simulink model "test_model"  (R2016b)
settings: Solver=VariableStepAuto  StartTime=0.0  StopTime=8.4  RelTol=1e-3
InitFcn:
  | clear mex
  | delete test_model_sfun.mexw64
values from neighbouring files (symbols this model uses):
  g = 9.81    [modelParameters.m]    (also in analyzeIMU_data.m = 9.8; getMomentOfInertia.m = 9.80665)
  height_controlled_o = (((Rm*If +      + (((omega_o * 2 * Rm * Kv * Kq       * Kd + 1)^2) - 1)/(4* Rm*Kv^2*Kq      *Kd))/Vb)*(Pmax- Pmin)+Pmin)    [modelParameters.m]
  If = 0.511    [modelParameters.m]    (also in thrustDragConstantCalculations.m = [If0; If1; If2; If3]; Kd_error.m = I_0 * sign(rotor_speed_0) + I_1 * rotor_speed_0 + I_2 * roto)
  Jreq = 4.2012e-05    [modelParameters.m]
  Jxx = 0.0130    (= 0.013)    [modelParameters.m]
  Jyy = 0.0140    (= 0.014)    [modelParameters.m]
  Jzz = 0.0285    [modelParameters.m]
  Kd = 1.0317e-7    (= 1.0317e-07)    [modelParameters.m]    (also in calcDragConstant.m = ((A'*A)^-1)*A'*b; thrustDragConstantCalculations.m = calcDragConstant(data, Pmin, Pmax, Rm, Kv, Kq, If); Kd_error.m)
  Kq = 96.3422    [modelParameters.m]    (also in thrustDragConstantCalculations.m; Kd_error.m)
  Kt = 8.6519e-6    (= 8.6519e-06)    [modelParameters.m]    (also in calcThrustConstant.m = ((A'*A)^(-1))*(A'*T); thrustDragConstantCalculations.m = calcThrustConstant(data))
  Kv = 96.3422    [modelParameters.m]    (also in thrustDragConstantCalculations.m; Kd_error.m)
  logAnalysisToggle = 1    [modelParameters.m]
  m = 1.244    [modelParameters.m]
  omega_o = sqrt((m*g)/(4*Kt))    [modelParameters.m]
  Pmax = 2e5    (= 200000)    [modelParameters.m]    (also in thrustDragConstantCalculations.m; Kd_error.m)
  Pmin = 1e5    (= 100000)    [modelParameters.m]    (also in thrustDragConstantCalculations.m; Kd_error.m)
  rhx = 0.16    [modelParameters.m]
  rhy = 0.16    [modelParameters.m]
  rhz = 0.03    [modelParameters.m]
  Rm = 0.2308    [modelParameters.m]    (also in thrustDragConstantCalculations.m; Kd_error.m)
  Tc = 0.04    [modelParameters.m]
  Tq = 0.005    [modelParameters.m]
  Vb = 11.1    [modelParameters.m]    (also in calcDragConstant.m = [data.(6); data.(6); data.(6); data.(6)]; Kd_error.m = data.(6))
  x_controlled_o = 0    [modelParameters.m]
  y_controlled_o = 0    [modelParameters.m]
  yaw_controlled_o = 0    [modelParameters.m]
undefined symbols (not defined in the file or in its folder): DiscIntNeverNeededParam
libraries: simulink x13, vrlib x2

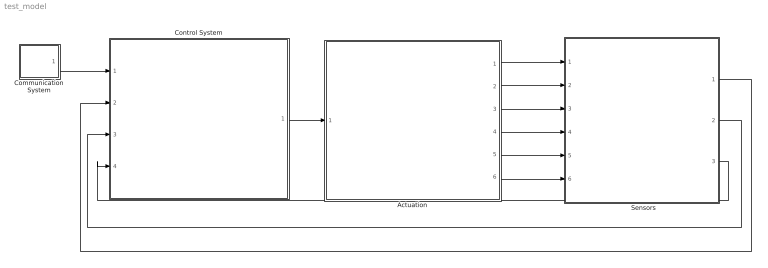
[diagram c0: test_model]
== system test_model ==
  "     Sensors   " : Subsystem
  Actuation : Subsystem
  Communication System : Subsystem
  Control System : Subsystem
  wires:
  Control System/1(P) -> Actuation/1(P)
  Communication System/1(setpoints) -> Control System/1(setpoints)
  Actuation/1(B_omega) -> "     Sensors   "/1(B_Omega)
  Actuation/2(euler_angles) -> "     Sensors   "/2(euler_angles)
  Actuation/3(B_vo) -> "     Sensors   "/3(B_vo)
  Actuation/4(E_ro) -> "     Sensors   "/4(E_ro)
  Actuation/5(B_vo_dot) -> "     Sensors   "/5(B_vo_dot)
  Actuation/6(B_g) -> "     Sensors   "/6(B_g)
  "     Sensors   "/3(current_position) -> Control System/4(current_position)
  "     Sensors   "/2(euler_rates) -> Control System/3(euler_rates)
  "     Sensors   "/1(euler_angles_filtered) -> Control System/2(euler_angles_filtered)

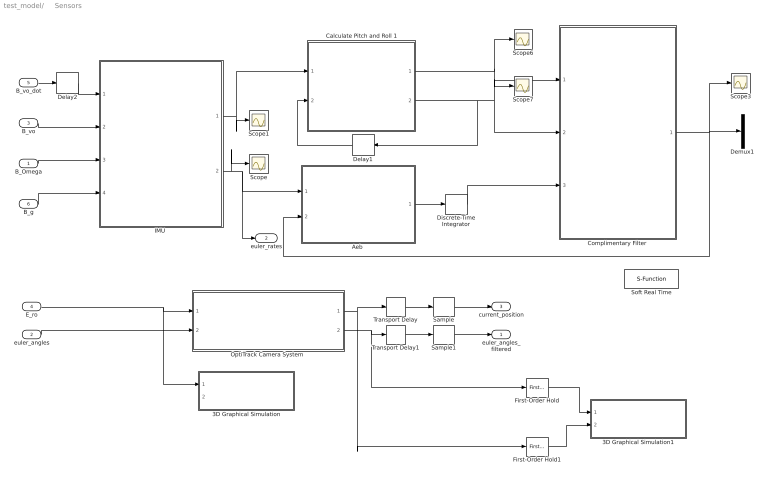
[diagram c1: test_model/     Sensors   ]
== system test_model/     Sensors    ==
  B_Omega : Inport
  euler_angles : Inport  Port=2
  B_vo : Inport  Port=3
  E_ro : Inport  Port=4
  B_vo_dot : Inport  Port=5
  B_g : Inport  Port=6
  3D Graphical Simulation : Subsystem  Commented=on
  3D Graphical Simulation1 : Subsystem  Commented=on
  "Aeb " : MATLAB Function  TreatAsAtomicUnit=on
  Calculate Pitch and Roll 1 : MATLAB Function  TreatAsAtomicUnit=on
  "Complimentary Filter " : MATLAB Function  TreatAsAtomicUnit=on
  Delay1 : Delay  DelayLength=1  InitialCondition=0  SampleTime=Tq
  Delay2 : Delay  DelayLength=1  InitialCondition=0  SampleTime=Tq
  Demux1 : Demux  Outputs=2
  Discrete-Time Integrator : DiscreteIntegrator  InitialConditionSetting=State (most efficient)  SampleTime=Tq  ICPrevOutput=DiscIntNeverNeededParam  ICPrevScaledInput=DiscIntNeverNeededParam
  First-Order Hold : simulink/Discrete/First-Order Hold  DisableCoverage=on  Ts=5e-3
  First-Order Hold1 : simulink/Discrete/First-Order Hold  DisableCoverage=on  Ts=5e-3
  "IMU " : Subsystem
  "OptiTrack Camera System " : Subsystem
  Sample : ZeroOrderHold  SampleTime=Tc
  Sample1 : ZeroOrderHold  SampleTime=Tc
  Scope{,1,3,6..7} (5 alike) : Scope
  Soft Real Time : S-Function  Commented=on  FunctionName=sfun_time  Parameters=x  SFunctionDeploymentMode=off  EnableBusSupport=off
  Transport Delay : TransportDelay  DelayTime=6e-3
  Transport Delay1 : TransportDelay  DelayTime=6e-3
  euler_angles_filtered : Outport
  euler_rates : Outport  Port=2
  current_position : Outport  Port=3
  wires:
  "IMU "/1(accelerometer) -> Calculate Pitch and Roll 1/1(accel_reading), Scope1/1
  "IMU "/2(gyroscope) -> Scope/1, euler_rates/1, "Aeb "/1(gyro_reading)
  B_vo/1 -> "IMU "/2(B_vo)
  B_Omega/1 -> "IMU "/3(B_Omega)
  B_g/1 -> "IMU "/4(B_g)
  Calculate Pitch and Roll 1/2(accel_roll) -> Scope7/1, "Complimentary Filter "/2(accel_roll), Delay1/1
  Calculate Pitch and Roll 1/1(accel_pitch) -> Scope6/1, "Complimentary Filter "/1(accel_pitch)
  Delay1/1 -> Calculate Pitch and Roll 1/2(accel_roll_prev)
  euler_angles/1 -> "OptiTrack Camera System "/2(yaw)
  First-Order Hold/1 -> 3D Graphical Simulation1/1("Euler Angles ")
  E_ro/1 -> 3D Graphical Simulation/1(Displacement), "OptiTrack Camera System "/1(E_ro)
  First-Order Hold1/1 -> 3D Graphical Simulation1/2(Displacement)
  B_vo_dot/1 -> Delay2/1
  Delay2/1 -> "IMU "/1(B_vo_dot)
  "Aeb "/1(euler_rates_IMU) -> Discrete-Time Integrator/1
  Discrete-Time Integrator/1 -> "Complimentary Filter "/3(euler_angles_gyro)
  "OptiTrack Camera System "/1(E_ro_camera) -> Transport Delay/1, First-Order Hold1/1
  "OptiTrack Camera System "/2(yaw_camera) -> First-Order Hold/1, Transport Delay1/1
  Transport Delay/1 -> Sample/1
  Transport Delay1/1 -> Sample1/1
  Sample/1 -> current_position/1
  Sample1/1 -> euler_angles_filtered/1
  "Complimentary Filter "/1(euler_angles_IMU) -> "Aeb "/2(euler_angles_IMU), Scope3/1, Demux1/1

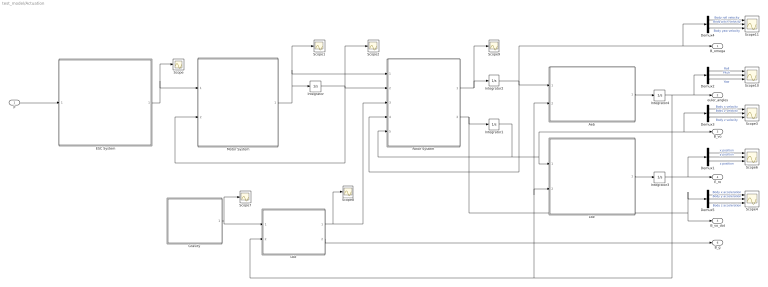
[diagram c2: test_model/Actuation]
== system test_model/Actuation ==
  P : Inport
  "Aeb " : MATLAB Function  TreatAsAtomicUnit=on
  Demux{1..5} (5 alike) : Demux  Outputs=3
  ESC System : MATLAB Function  TreatAsAtomicUnit=on
  "Gravity " : MATLAB Function  TreatAsAtomicUnit=on
  Integrator : Integrator  InitialCondition=[omega_o, omega_o, omega_o, omega_o]
  Integrator1 : Integrator  InitialCondition=[0; 0; 0]
  Integrator2 : Integrator  InitialCondition=[0; 0; 0]
  Integrator3 : Integrator  InitialCondition=[0; 0; 0]
  Integrator4 : Integrator  InitialCondition=[0; 0; 0]  ContinuousStateAttributes=['phi' 'theta' 'psi']
  "Lbe " : MATLAB Function  TreatAsAtomicUnit=on
  "Lbe " : MATLAB Function  TreatAsAtomicUnit=on
  Motor System : MATLAB Function  TreatAsAtomicUnit=on
  "Rotor System " : MATLAB Function  TreatAsAtomicUnit=on
  Scope{,1..2,7..9} (6 alike) : Scope
  Scope{3..4,6,10..11} (5 alike) : Scope  NumInputPorts=3
  B_omega : Outport
  euler_angles : Outport  Port=2
  B_vo : Outport  Port=3
  E_ro : Outport  Port=4
  B_vo_dot : Outport  Port=5
  B_g : Outport  Port=6
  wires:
  ESC System/1(Vb_eff) -> Scope/1, Motor System/1(Vb_eff)
  Motor System/1(w_dot) -> Integrator/1, "Rotor System "/1(w_dot), Scope1/1
  Integrator/1 -> Motor System/2(w), "Rotor System "/2(w), Scope2/1
  "Rotor System "/1(B_omega_dot) -> Scope9/1, Integrator2/1
  Integrator2/1 -> "Rotor System "/4(B_omega), B_omega/1, Demux4/1, "Aeb "/1(B_omega)
  "Aeb "/1(euler_rates) -> Integrator4/1
  "Gravity "/1(E_Fg) -> Scope7/1, "Lbe "/1(E_Fg)
  "Lbe "/1(E_ro) -> Integrator3/1
  Integrator3/1 -> Demux1/1, E_ro/1
  "Lbe "/1(B_Fg) -> Scope8/1, "Rotor System "/3(B_Fg)
  "Lbe "/2(B_g) -> B_g/1
  Demux1/2 -> Scope6/2  "y position"
  Demux1/1 -> Scope6/1  "x position"
  Demux1/3 -> Scope6/3  "z position"
  Demux2/2 -> Scope10/2  "Pitch"
  Demux2/1 -> Scope10/1  "Roll"
  Demux2/3 -> Scope10/3  "Yaw"
  Demux4/2 -> Scope11/2  "Body pitch velocity"
  Demux4/1 -> Scope11/1  "Body roll velocity"
  Demux4/3 -> Scope11/3  "Body yaw velocity"
  Demux3/2 -> Scope3/2  "Body y velocity"
  Demux3/1 -> Scope3/1  "Body x velocity"
  Demux3/3 -> Scope3/3  "Body z velocity"
  Demux5/2 -> Scope4/2  "Body y acceleration"
  Demux5/1 -> Scope4/1  "Body x acceleration"
  Demux5/3 -> Scope4/3  "Body z acceleration"
  Integrator1/1 -> "Rotor System "/5(B_vo), "Lbe "/1(B_vo), Demux3/1, B_vo/1
  "Rotor System "/2(B_vo_dot) -> Demux5/1, B_vo_dot/1, Integrator1/1
  Integrator4/1 -> euler_angles/1, Demux2/1, "Lbe "/2(euler_angles), "Aeb "/2(euler_angles), "Lbe "/2(euler_angles)
  P/1 -> ESC System/1(P)

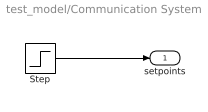
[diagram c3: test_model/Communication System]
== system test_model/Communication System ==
  Step : Step  Before=[0; 0; 0; 0]  After=[1; 1; 0; 0]  SampleTime=Tq
  setpoints : Outport
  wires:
  Step/1 -> setpoints/1

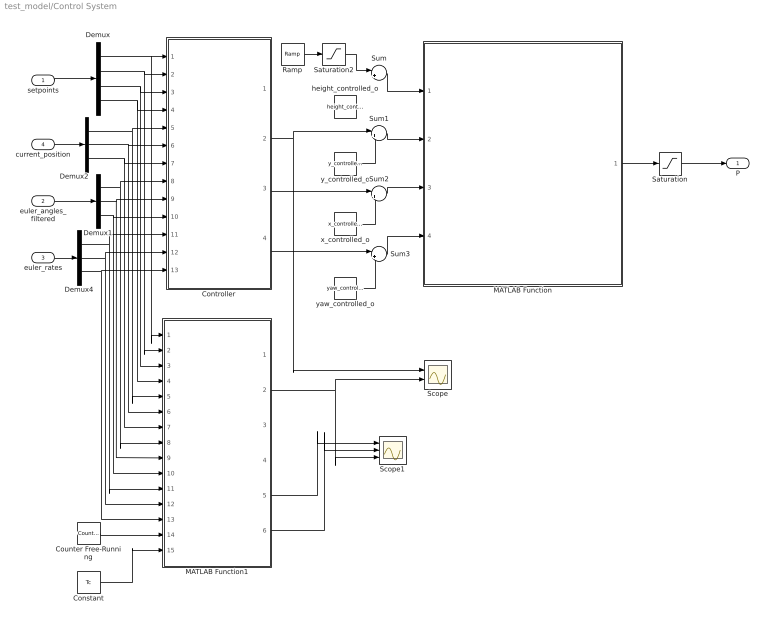
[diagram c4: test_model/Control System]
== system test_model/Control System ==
  setpoints : Inport
  euler_angles_filtered : Inport  Port=2
  euler_rates : Inport  Port=3
  current_position : Inport  Port=4
  Constant : Constant  Value=Tc  SampleTime=Tc
  Controller : Subsystem
  Counter Free-Running : simulink/Sources/Counter Free-Running  NumBits=32  tsamp=Tc
  Demux : Demux
  Demux1 : Demux  Outputs=3
  Demux2 : Demux  Outputs=3
  Demux4 : Demux  Outputs=3
  MATLAB Function : MATLAB Function  TreatAsAtomicUnit=on
  MATLAB Function1 : MATLAB Function  TreatAsAtomicUnit=on  SystemSampleTime=Tq
  Ramp : simulink/Sources/Ramp  slope=height_controlled_o  start=6.32  X0=0
  Saturation : Saturate  UpperLimit=Pmax*ones(4,1)  LowerLimit=Pmin*ones(4,1)
  Saturation2 : Saturate  UpperLimit=height_controlled_o  LowerLimit=0
  Scope : Scope  NumInputPorts=2
  Scope1 : Scope  NumInputPorts=3
  Sum{,1..3} (4 alike) : Sum  Inputs=|++
  height_controlled_o : Constant  Value=height_controlled_o  SampleTime=Tc
  x_controlled_o : Constant  Value=x_controlled_o
  y_controlled_o : Constant  Value=y_controlled_o
  yaw_controlled_o : Constant  Value=yaw_controlled_o
  P : Outport
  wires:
  setpoints/1 -> Demux/1
  euler_angles_filtered/1 -> Demux1/1
  current_position/1 -> Demux2/1
  euler_rates/1 -> Demux4/1
  Demux/1 -> MATLAB Function1/1(set_x), Controller/1(x_setpoint)
  Demux/2 -> MATLAB Function1/2(set_y), Controller/2(y_setpoint)
  Demux/3 -> MATLAB Function1/3(set_z), Controller/3(z_setpoint)
  Demux2/1 -> MATLAB Function1/5(cur_x), Controller/5(x_position)
  Demux2/2 -> Controller/6(y_position), MATLAB Function1/6(cur_y)
  Demux2/3 -> MATLAB Function1/7(cur_z), Controller/7(z_position)
  Controller/2(y_controlled) -> Scope/1, Sum1/1
  Controller/4(yaw_controlled) -> Sum3/1
  y_controlled_o/1 -> Sum1/2
  x_controlled_o/1 -> Sum2/2
  yaw_controlled_o/1 -> Sum3/2
  MATLAB Function/1(P) -> Saturation/1
  Demux1/1 -> Controller/8(roll), MATLAB Function1/8(cur_phi)
  Demux1/2 -> MATLAB Function1/9(cur_theta), Controller/9(pitch)
  Demux4/1 -> Controller/11(roll_rate), MATLAB Function1/11(cur_phi_d)
  Demux4/2 -> Controller/12(pitch_rate), MATLAB Function1/12(cur_theta_d)
  Demux4/3 -> MATLAB Function1/13(cur_psi_d), Controller/13(yaw_rate)
  Demux/4 -> MATLAB Function1/4(set_yaw), Controller/4(yaw_setpoint)
  Demux1/3 -> MATLAB Function1/10(cur_psi), Controller/10(yaw)
  Controller/3(x_controlled) -> Sum2/1
  Counter Free-Running/1 -> MATLAB Function1/14(vrpn_id)
  Saturation/1 -> P/1
  Constant/1 -> MATLAB Function1/15(Tc)
  Sum3/1 -> MATLAB Function/4(yaw_controlled)
  Sum2/1 -> MATLAB Function/3(x_controlled)
  Sum1/1 -> MATLAB Function/2(y_controlled)
  Sum/1 -> MATLAB Function/1(height_controlled)
  MATLAB Function1/5(pid_y_out) -> Scope1/1
  MATLAB Function1/6(pid_roll_out) -> Scope1/2
  MATLAB Function1/2(y_cor) -> Scope1/3, Scope/2
  Saturation2/1 -> Sum/1
  Ramp/1 -> Saturation2/1

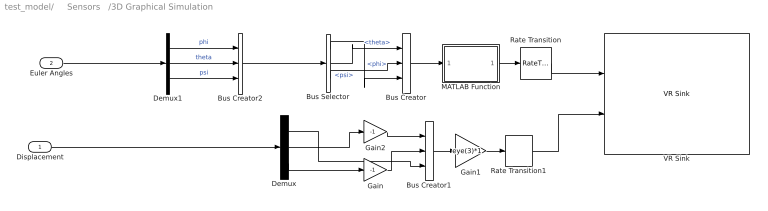
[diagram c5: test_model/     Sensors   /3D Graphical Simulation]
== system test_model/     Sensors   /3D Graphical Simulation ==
  Displacement : Inport
  Euler Angles : Inport  Port=2
  Bus Creator : BusCreator  Inputs=3
  Bus Creator1 : BusCreator  Inputs=3
  Bus Creator2 : BusCreator  Inputs=3
  Bus Selector : BusSelector  OutputSignals=phi,theta,psi
  Demux : Demux  Outputs=3
  Demux1 : Demux  Outputs=3
  Gain : Gain  Gain=-1
  Gain1 : Gain  Gain=eye(3)*1  Multiplication=Matrix(K*u)
  Gain2 : Gain  Gain=-1
  MATLAB Function : MATLAB Function  TreatAsAtomicUnit=on
  Rate Transition : RateTransition  OutPortSampleTime=0.06
  Rate Transition1 : RateTransition  OutPortSampleTime=0.06
  VR Sink : vrlib/VR Sink  InstantiateOnLoad=on  SampleTime=-1  ViewEnable=on  RemoteChange=off  RemoteView=off  FieldsWritten=Helicopter.rotation.4.1.1.double#Helicopter.translation.3.1.1.double  WorldFileName=quadrotor_world_ucart.wrl  AutoView=on  VideoDimensions=[]  AllowVariableSize=off
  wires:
  Displacement/1 -> Demux/1
  Bus Creator2/1 -> Bus Selector/1
  Demux/1 -> Bus Creator1/3
  Gain/1 -> Bus Creator1/2
  Gain2/1 -> Bus Creator1/1
  Rate Transition1/1 -> VR Sink/2
  Rate Transition/1 -> VR Sink/1
  Demux/3 -> Gain/1
  Demux/2 -> Gain2/1
  Bus Creator1/1 -> Gain1/1
  Bus Selector/1 -> Bus Creator/3  "<phi>"
  Bus Selector/3 -> Bus Creator/2  "<psi>"
  Bus Selector/2 -> Bus Creator/1  "<theta>"
  Gain1/1 -> Rate Transition1/1
  Demux1/3 -> Bus Creator2/3  "psi"
  Demux1/2 -> Bus Creator2/2  "theta"
  Demux1/1 -> Bus Creator2/1  "phi"
  Euler Angles/1 -> Demux1/1
  Bus Creator/1 -> MATLAB Function/1(u)
  MATLAB Function/1(y) -> Rate Transition/1

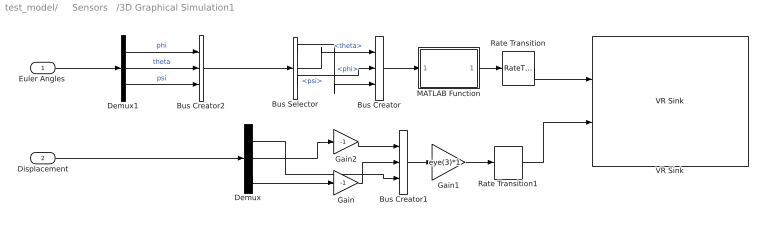
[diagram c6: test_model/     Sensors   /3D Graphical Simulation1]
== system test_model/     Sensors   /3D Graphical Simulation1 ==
  "Euler Angles " : Inport
  Displacement : Inport  Port=2
  Bus Creator : BusCreator  Inputs=3
  Bus Creator1 : BusCreator  Inputs=3
  Bus Creator2 : BusCreator  Inputs=3
  Bus Selector : BusSelector  OutputSignals=phi,theta,psi
  Demux : Demux  Outputs=3
  Demux1 : Demux  Outputs=3
  Gain : Gain  Gain=-1
  Gain1 : Gain  Gain=eye(3)*1  Multiplication=Matrix(K*u)
  Gain2 : Gain  Gain=-1
  MATLAB Function : MATLAB Function  TreatAsAtomicUnit=on
  Rate Transition : RateTransition  OutPortSampleTime=0.06
  Rate Transition1 : RateTransition  OutPortSampleTime=0.06
  VR Sink : vrlib/VR Sink  InstantiateOnLoad=on  SampleTime=-1  ViewEnable=on  RemoteChange=off  RemoteView=off  FieldsWritten=Helicopter.rotation.4.1.1.double#Helicopter.translation.3.1.1.double  WorldFileName=quadrotor_world_ucart.wrl  AutoView=on  VideoDimensions=[]  AllowVariableSize=off
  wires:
  Bus Creator2/1 -> Bus Selector/1
  Demux/1 -> Bus Creator1/3
  Gain/1 -> Bus Creator1/2
  Gain2/1 -> Bus Creator1/1
  Rate Transition1/1 -> VR Sink/2
  Rate Transition/1 -> VR Sink/1
  Demux/3 -> Gain/1
  Demux/2 -> Gain2/1
  Bus Creator1/1 -> Gain1/1
  Bus Selector/1 -> Bus Creator/3  "<phi>"
  Bus Selector/3 -> Bus Creator/2  "<psi>"
  Bus Selector/2 -> Bus Creator/1  "<theta>"
  Gain1/1 -> Rate Transition1/1
  Demux1/3 -> Bus Creator2/3  "psi"
  Demux1/2 -> Bus Creator2/2  "theta"
  Demux1/1 -> Bus Creator2/1  "phi"
  Bus Creator/1 -> MATLAB Function/1(u)
  MATLAB Function/1(y) -> Rate Transition/1
  Displacement/1 -> Demux/1
  "Euler Angles "/1 -> Demux1/1

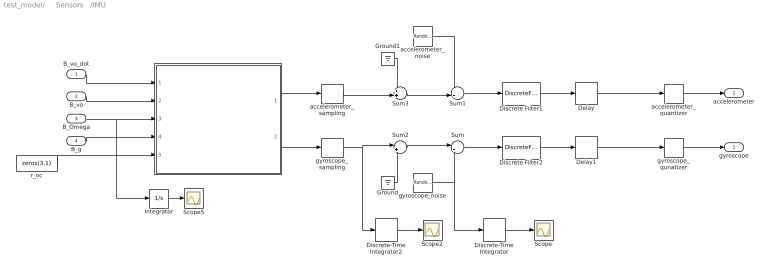
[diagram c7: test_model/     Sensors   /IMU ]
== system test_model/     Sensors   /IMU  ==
  B_vo_dot : Inport
  B_vo : Inport  Port=2
  B_Omega : Inport  Port=3
  B_g : Inport  Port=4
  " " : MATLAB Function  TreatAsAtomicUnit=on
  Delay : Delay  DelayLength=4  InitialCondition=0  SampleTime=Tq
  Delay1 : Delay  DelayLength=4  InitialCondition=0  SampleTime=Tq
  Discrete Filter1 : DiscreteFilter  Numerator=[0 0.1454]  Denominator=[1 -0.8546]  SampleTime=Tq
  Discrete Filter2 : DiscreteFilter  Numerator=[0 0.1454]  Denominator=[1 -0.8546]  SampleTime=Tq
  Discrete-Time Integrator : DiscreteIntegrator  InitialConditionSetting=State (most efficient)  SampleTime=-1  ICPrevOutput=DiscIntNeverNeededParam  ICPrevScaledInput=DiscIntNeverNeededParam
  Discrete-Time Integrator2 : DiscreteIntegrator  InitialConditionSetting=State (most efficient)  SampleTime=-1  ICPrevOutput=DiscIntNeverNeededParam  ICPrevScaledInput=DiscIntNeverNeededParam
  Ground : Ground
  Ground1 : Ground
  Integrator : Integrator
  Scope : Scope
  Scope2 : Scope
  Scope5 : Scope
  Sum : Sum  Inputs=|++
  Sum1 : Sum  Inputs=++|
  Sum2 : Sum  Inputs=|++
  Sum3 : Sum  Inputs=++|
  accelerometer_noise : RandomNumber  Mean=zeros(3,1)  Variance=[ 3e-7 ; 3.3e-7 ; 7.2e-7 ]  Seed=[0,1,2]  SampleTime=Tq
  accelerometer_quantizer : Quantizer  QuantizationInterval=2.4400e-04
  accelerometer_sampling : ZeroOrderHold  SampleTime=Tq
  gyroscope_noise : RandomNumber  Mean=zeros(3,1)  Variance=[ 2.2e-8 ; 1.1e-7 ; 2.4e-8 ]  Seed=[0,1,2]  SampleTime=Tq
  gyroscope_qunatizer : Quantizer  QuantizationInterval=1.1e-3
  gyroscope_sampling : ZeroOrderHold  SampleTime=Tq
  r_oc : Constant  Value=zeros(3,1)
  accelerometer : Outport
  gyroscope : Outport  Port=2
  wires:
  accelerometer_noise/1 -> Sum1/1
  Sum/1 -> Discrete Filter2/1
  Sum2/1 -> Sum/1
  Sum3/1 -> Sum1/2
  gyroscope_noise/1 -> Sum/2, Discrete-Time Integrator/1
  Sum1/1 -> Discrete Filter1/1
  gyroscope_sampling/1 -> Sum2/1, Discrete-Time Integrator2/1
  accelerometer_sampling/1 -> Sum3/2
  Ground/1 -> Sum2/2
  Ground1/1 -> Sum3/1
  B_vo_dot/1 -> " "/1(B_vo_dot)
  B_vo/1 -> " "/2(B_vo)
  B_Omega/1 -> Integrator/1, " "/3(B_Omega)
  B_g/1 -> " "/4(B_g)
  r_oc/1 -> " "/5(r_oc)
  " "/2(gyroReading) -> gyroscope_sampling/1
  " "/1(accelReading) -> accelerometer_sampling/1
  Discrete-Time Integrator/1 -> Scope/1
  Discrete-Time Integrator2/1 -> Scope2/1
  Integrator/1 -> Scope5/1
  gyroscope_qunatizer/1 -> gyroscope/1
  accelerometer_quantizer/1 -> accelerometer/1
  Discrete Filter2/1 -> Delay1/1
  Discrete Filter1/1 -> Delay/1
  Delay/1 -> accelerometer_quantizer/1
  Delay1/1 -> gyroscope_qunatizer/1

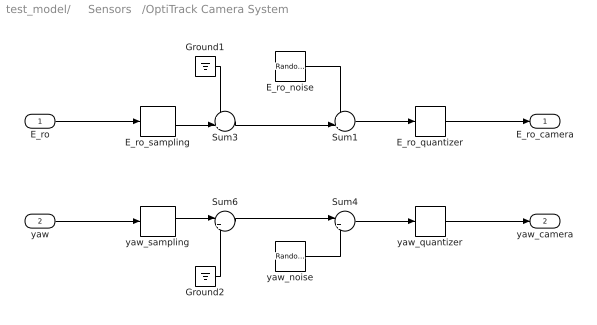
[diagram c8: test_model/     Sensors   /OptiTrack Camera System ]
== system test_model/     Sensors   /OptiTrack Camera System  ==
  E_ro : Inport
  yaw : Inport  Port=2
  E_ro_noise : RandomNumber  Mean=zeros(3,1)  Variance=[ 7.9664e-10 ; 1.1928e-10 ; 5.0636e-10 ]  Seed=[0,1,2]  SampleTime=Tc
  E_ro_quantizer : Quantizer  QuantizationInterval=2.4400e-04
  E_ro_sampling : ZeroOrderHold  SampleTime=Tc
  Ground1 : Ground
  Ground2 : Ground
  Sum1 : Sum  Inputs=++|
  Sum3 : Sum  Inputs=++|
  Sum4 : Sum  Inputs=|++
  Sum6 : Sum  Inputs=|++
  yaw_noise : RandomNumber  Variance=1.0783e-9  SampleTime=Tc
  yaw_quantizer : Quantizer  QuantizationInterval=1.1e-3
  yaw_sampling : ZeroOrderHold  SampleTime=Tc
  E_ro_camera : Outport
  yaw_camera : Outport  Port=2
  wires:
  E_ro_noise/1 -> Sum1/1
  Sum3/1 -> Sum1/2
  Sum1/1 -> E_ro_quantizer/1
  E_ro_sampling/1 -> Sum3/2
  Ground1/1 -> Sum3/1
  Sum4/1 -> yaw_quantizer/1
  Sum6/1 -> Sum4/1
  yaw_noise/1 -> Sum4/2
  yaw_sampling/1 -> Sum6/1
  Ground2/1 -> Sum6/2
  yaw/1 -> yaw_sampling/1
  E_ro/1 -> E_ro_sampling/1
  E_ro_quantizer/1 -> E_ro_camera/1
  yaw_quantizer/1 -> yaw_camera/1

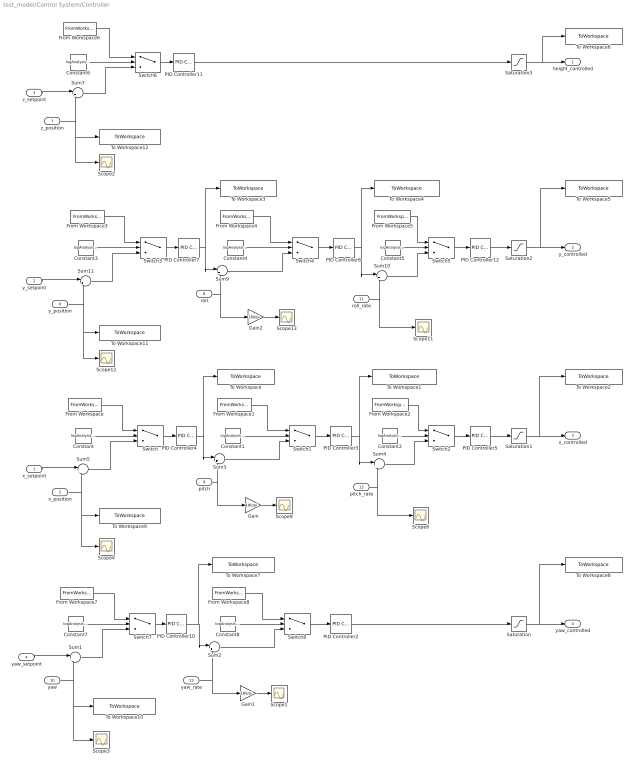
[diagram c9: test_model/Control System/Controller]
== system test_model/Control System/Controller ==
  x_setpoint : Inport
  y_setpoint : Inport  Port=2
  z_setpoint : Inport  Port=3
  yaw_setpoint : Inport  Port=4
  x_position : Inport  Port=5
  y_position : Inport  Port=6
  z_position : Inport  Port=7
  roll : Inport  Port=8
  pitch : Inport  Port=9
  yaw : Inport  Port=10
  roll_rate : Inport  Port=11
  pitch_rate : Inport  Port=12
  yaw_rate : Inport  Port=13
  Constant{,1..8} (9 alike) : Constant  Value=logAnalysisToggle
  From Workspace : FromWorkspace  VariableName=x_error  SampleTime=Tc
  From Workspace1 : FromWorkspace  VariableName=pitch_error  SampleTime=Tc
  From Workspace2 : FromWorkspace  VariableName=pitchrate_error  SampleTime=Tq
  From Workspace3 : FromWorkspace  VariableName=y_error  SampleTime=Tc
  From Workspace4 : FromWorkspace  VariableName=roll_error  SampleTime=Tc
  From Workspace5 : FromWorkspace  VariableName=rollrate_error  SampleTime=Tq
  From Workspace6 : FromWorkspace  VariableName=z_error  SampleTime=Tc
  From Workspace7 : FromWorkspace  VariableName=yaw_error  SampleTime=Tc
  From Workspace8 : FromWorkspace  VariableName=yawrate_error  SampleTime=Tc
  Gain : Gain  Gain=180/pi
  Gain1 : Gain  Gain=180/pi
  Gain2 : Gain  Gain=180/pi
  PID Controller10 : simulink/Continuous/PID Controller  Controller=PD  TimeDomain=Discrete-time  SampleTime=Tc  IntegratorMethod=Forward Euler  FilterMethod=Forward Euler  Form=Parallel  UseFilter=on  ControllerParametersSource=internal  P=4.73868196952772  I=2.36803176515497  D=1.0129554639517  N=3.83298618768959  InitialConditionSource=internal  InitialConditionForIntegrator=0  InitialConditionForFilter=0  ExternalReset=none  LimitOutput=off  UpperSaturationLimit=inf  LowerSaturationLimit=-inf  LinearizeAsGain=on  AntiWindupMode=none  Kb=1  TrackingMode=off  Kt=1  PParamMin=[]  PParamMax=[]  IParamMin=[]  IParamMax=[]  DParamMin=[]  DParamMax=[]  NParamMin=[]  NParamMax=[]  KbParamMin=[]  KbParamMax=[]  KtParamMin=[]  KtParamMax=[]  POutMin=[]  POutMax=[]  IOutMin=[]  IOutMax=[]  DOutMin=[]  DOutMax=[]  NOutMin=[]  NOutMax=[]  KbOutMin=[]  KbOutMax=[]  KtOutMin=[]  KtOutMax=[]  IntegratorOutMin=[]  IntegratorOutMax=[]  FilterOutMin=[]  FilterOutMax=[]  SumOutMin=[]  SumOutMax=[]  SumI1OutMin=[]  SumI1OutMax=[]  SumI2OutMin=[]  SumI2OutMax=[]  SumI3OutMin=[]  SumI3OutMax=[]  SumDOutMin=[]  SumDOutMax=[]  SaturationOutMin=[]  SaturationOutMax=[]  IntegratorContinuousStateAttributes=''  IntegratorStateMustResolveToSignalObject=off  IntegratorRTWStateStorageClass=Auto  FilterContinuousStateAttributes=''  FilterStateMustResolveToSignalObject=off  FilterRTWStateStorageClass=Auto  DifferentiatorICPrevScaledInput=0  DifferentiatorOutMin=[]  DifferentiatorOutMax=[]
  PID Controller11 : simulink/Continuous/PID Controller  Controller=PID  TimeDomain=Discrete-time  SampleTime=Tc  IntegratorMethod=Forward Euler  FilterMethod=Forward Euler  Form=Parallel  UseFilter=off  ControllerParametersSource=internal  P=-3138.91816077077  I=-320.189162634817  D=-7421.98260028101  N=5.79502261645411  InitialConditionSource=internal  InitialConditionForIntegrator=0  InitialConditionForFilter=0  ExternalReset=none  LimitOutput=off  UpperSaturationLimit=inf  LowerSaturationLimit=-inf  LinearizeAsGain=on  AntiWindupMode=none  Kb=1  TrackingMode=off  Kt=1  PParamMin=[]  PParamMax=[]  IParamMin=[]  IParamMax=[]  DParamMin=[]  DParamMax=[]  NParamMin=[]  NParamMax=[]  KbParamMin=[]  KbParamMax=[]  KtParamMin=[]  KtParamMax=[]  POutMin=[]  POutMax=[]  IOutMin=[]  IOutMax=[]  DOutMin=[]  DOutMax=[]  NOutMin=[]  NOutMax=[]  KbOutMin=[]  KbOutMax=[]  KtOutMin=[]  KtOutMax=[]  IntegratorOutMin=[]  IntegratorOutMax=[]  FilterOutMin=[]  FilterOutMax=[]  SumOutMin=[]  SumOutMax=[]  SumI1OutMin=[]  SumI1OutMax=[]  SumI2OutMin=[]  SumI2OutMax=[]  SumI3OutMin=[]  SumI3OutMax=[]  SumDOutMin=[]  SumDOutMax=[]  SaturationOutMin=[]  SaturationOutMax=[]  IntegratorContinuousStateAttributes=''  IntegratorStateMustResolveToSignalObject=off  IntegratorRTWStateStorageClass=Auto  FilterContinuousStateAttributes=''  FilterStateMustResolveToSignalObject=off  FilterRTWStateStorageClass=Auto  DifferentiatorICPrevScaledInput=0  DifferentiatorOutMin=[]  DifferentiatorOutMax=[]
  PID Controller12 : simulink/Continuous/PID Controller  Controller=P  TimeDomain=Discrete-time  SampleTime=Tq  IntegratorMethod=Forward Euler  FilterMethod=Forward Euler  Form=Parallel  UseFilter=off  ControllerParametersSource=internal  P=1835.12180866282  I=1575.82088970639  D=550  N=244.660686071579  InitialConditionSource=internal  InitialConditionForIntegrator=0  InitialConditionForFilter=0  ExternalReset=none  LimitOutput=off  UpperSaturationLimit=inf  LowerSaturationLimit=-inf  LinearizeAsGain=on  AntiWindupMode=none  Kb=1  TrackingMode=off  Kt=1  PParamMin=[]  PParamMax=[]  IParamMin=[]  IParamMax=[]  DParamMin=[]  DParamMax=[]  NParamMin=[]  NParamMax=[]  KbParamMin=[]  KbParamMax=[]  KtParamMin=[]  KtParamMax=[]  POutMin=[]  POutMax=[]  IOutMin=[]  IOutMax=[]  DOutMin=[]  DOutMax=[]  NOutMin=[]  NOutMax=[]  KbOutMin=[]  KbOutMax=[]  KtOutMin=[]  KtOutMax=[]  IntegratorOutMin=[]  IntegratorOutMax=[]  FilterOutMin=[]  FilterOutMax=[]  SumOutMin=[]  SumOutMax=[]  SumI1OutMin=[]  SumI1OutMax=[]  SumI2OutMin=[]  SumI2OutMax=[]  SumI3OutMin=[]  SumI3OutMax=[]  SumDOutMin=[]  SumDOutMax=[]  SaturationOutMin=[]  SaturationOutMax=[]  IntegratorContinuousStateAttributes=''  IntegratorStateMustResolveToSignalObject=off  IntegratorRTWStateStorageClass=Auto  FilterContinuousStateAttributes=''  FilterStateMustResolveToSignalObject=off  FilterRTWStateStorageClass=Auto  DifferentiatorICPrevScaledInput=0  DifferentiatorOutMin=[]  DifferentiatorOutMax=[]
  PID Controller2 : simulink/Continuous/PID Controller  Controller=P  TimeDomain=Discrete-time  SampleTime=Tc  IntegratorMethod=Forward Euler  FilterMethod=Forward Euler  Form=Parallel  UseFilter=on  ControllerParametersSource=internal  P=10205.7985086303  I=-77.7  D=2.32  N=1/0.0818  InitialConditionSource=internal  InitialConditionForIntegrator=0  InitialConditionForFilter=0  ExternalReset=none  ZeroCross=off  LimitOutput=off  UpperSaturationLimit=inf  LowerSaturationLimit=-inf  LinearizeAsGain=on  AntiWindupMode=none  Kb=1  TrackingMode=off  Kt=1  PParamMin=[]  PParamMax=[]  IParamMin=[]  IParamMax=[]  DParamMin=[]  DParamMax=[]  NParamMin=[]  NParamMax=[]  KbParamMin=[]  KbParamMax=[]  KtParamMin=[]  KtParamMax=[]  POutMin=[]  POutMax=[]  IOutMin=[]  IOutMax=[]  DOutMin=[]  DOutMax=[]  NOutMin=[]  NOutMax=[]  KbOutMin=[]  KbOutMax=[]  KtOutMin=[]  KtOutMax=[]  IntegratorOutMin=[]  IntegratorOutMax=[]  FilterOutMin=[]  FilterOutMax=[]  SumOutMin=[]  SumOutMax=[]  SumI1OutMin=[]  SumI1OutMax=[]  SumI2OutMin=[]  SumI2OutMax=[]  SumI3OutMin=[]  SumI3OutMax=[]  SumDOutMin=[]  SumDOutMax=[]  SaturationOutMin=[]  SaturationOutMax=[]  IntegratorContinuousStateAttributes=''  IntegratorStateMustResolveToSignalObject=off  IntegratorRTWStateStorageClass=Auto  FilterContinuousStateAttributes=''  FilterStateMustResolveToSignalObject=off  FilterRTWStateStorageClass=Auto  DifferentiatorICPrevScaledInput=0  DifferentiatorOutMin=[]  DifferentiatorOutMax=[]
  PID Controller3 : simulink/Continuous/PID Controller  Controller=P  TimeDomain=Discrete-time  SampleTime=Tc  IntegratorMethod=Forward Euler  FilterMethod=Forward Euler  Form=Parallel  UseFilter=off  ControllerParametersSource=internal  P=1  I=35.1207902652377  D=0.2  N=40.0107970227961  InitialConditionSource=internal  InitialConditionForIntegrator=0  InitialConditionForFilter=0  ExternalReset=none  LimitOutput=off  UpperSaturationLimit=inf  LowerSaturationLimit=-inf  LinearizeAsGain=on  AntiWindupMode=none  Kb=1  TrackingMode=off  Kt=1  PParamMin=[]  PParamMax=[]  IParamMin=[]  IParamMax=[]  DParamMin=[]  DParamMax=[]  NParamMin=[]  NParamMax=[]  KbParamMin=[]  KbParamMax=[]  KtParamMin=[]  KtParamMax=[]  POutMin=[]  POutMax=[]  IOutMin=[]  IOutMax=[]  DOutMin=[]  DOutMax=[]  NOutMin=[]  NOutMax=[]  KbOutMin=[]  KbOutMax=[]  KtOutMin=[]  KtOutMax=[]  IntegratorOutMin=[]  IntegratorOutMax=[]  FilterOutMin=[]  FilterOutMax=[]  SumOutMin=[]  SumOutMax=[]  SumI1OutMin=[]  SumI1OutMax=[]  SumI2OutMin=[]  SumI2OutMax=[]  SumI3OutMin=[]  SumI3OutMax=[]  SumDOutMin=[]  SumDOutMax=[]  SaturationOutMin=[]  SaturationOutMax=[]  IntegratorContinuousStateAttributes=''  IntegratorStateMustResolveToSignalObject=off  IntegratorRTWStateStorageClass=Auto  FilterContinuousStateAttributes=''  FilterStateMustResolveToSignalObject=off  FilterRTWStateStorageClass=Auto  DifferentiatorICPrevScaledInput=0  DifferentiatorOutMin=[]  DifferentiatorOutMax=[]
  PID Controller4 : simulink/Continuous/PID Controller  Controller=PD  TimeDomain=Discrete-time  SampleTime=Tc  IntegratorMethod=Forward Euler  FilterMethod=Forward Euler  Form=Parallel  UseFilter=on  ControllerParametersSource=internal  P=-0.00239291827793903  I=0.005  D=-0.101936697537801  N=33.9318377685715  InitialConditionSource=internal  InitialConditionForIntegrator=0  InitialConditionForFilter=0  ExternalReset=none  LimitOutput=off  UpperSaturationLimit=inf  LowerSaturationLimit=-inf  LinearizeAsGain=on  AntiWindupMode=none  Kb=1  TrackingMode=off  Kt=1  PParamMin=[]  PParamMax=[]  IParamMin=[]  IParamMax=[]  DParamMin=[]  DParamMax=[]  NParamMin=[]  NParamMax=[]  KbParamMin=[]  KbParamMax=[]  KtParamMin=[]  KtParamMax=[]  POutMin=[]  POutMax=[]  IOutMin=[]  IOutMax=[]  DOutMin=[]  DOutMax=[]  NOutMin=[]  NOutMax=[]  KbOutMin=[]  KbOutMax=[]  KtOutMin=[]  KtOutMax=[]  IntegratorOutMin=[]  IntegratorOutMax=[]  FilterOutMin=[]  FilterOutMax=[]  SumOutMin=[]  SumOutMax=[]  SumI1OutMin=[]  SumI1OutMax=[]  SumI2OutMin=[]  SumI2OutMax=[]  SumI3OutMin=[]  SumI3OutMax=[]  SumDOutMin=[]  SumDOutMax=[]  SaturationOutMin=[]  SaturationOutMax=[]  IntegratorContinuousStateAttributes=''  IntegratorStateMustResolveToSignalObject=off  IntegratorRTWStateStorageClass=Auto  FilterContinuousStateAttributes=''  FilterStateMustResolveToSignalObject=off  FilterRTWStateStorageClass=Auto  DifferentiatorICPrevScaledInput=0  DifferentiatorOutMin=[]  DifferentiatorOutMax=[]
  PID Controller5 : simulink/Continuous/PID Controller  Controller=P  TimeDomain=Discrete-time  SampleTime=Tq  IntegratorMethod=Forward Euler  FilterMethod=Forward Euler  Form=Parallel  UseFilter=off  ControllerParametersSource=internal  P=1835.12180866282  I=1575.82088970639  D=550  N=244.660686071579  InitialConditionSource=internal  InitialConditionForIntegrator=0  InitialConditionForFilter=0  ExternalReset=none  LimitOutput=off  UpperSaturationLimit=inf  LowerSaturationLimit=-inf  LinearizeAsGain=on  AntiWindupMode=none  Kb=1  TrackingMode=off  Kt=1  PParamMin=[]  PParamMax=[]  IParamMin=[]  IParamMax=[]  DParamMin=[]  DParamMax=[]  NParamMin=[]  NParamMax=[]  KbParamMin=[]  KbParamMax=[]  KtParamMin=[]  KtParamMax=[]  POutMin=[]  POutMax=[]  IOutMin=[]  IOutMax=[]  DOutMin=[]  DOutMax=[]  NOutMin=[]  NOutMax=[]  KbOutMin=[]  KbOutMax=[]  KtOutMin=[]  KtOutMax=[]  IntegratorOutMin=[]  IntegratorOutMax=[]  FilterOutMin=[]  FilterOutMax=[]  SumOutMin=[]  SumOutMax=[]  SumI1OutMin=[]  SumI1OutMax=[]  SumI2OutMin=[]  SumI2OutMax=[]  SumI3OutMin=[]  SumI3OutMax=[]  SumDOutMin=[]  SumDOutMax=[]  SaturationOutMin=[]  SaturationOutMax=[]  IntegratorContinuousStateAttributes=''  IntegratorStateMustResolveToSignalObject=off  IntegratorRTWStateStorageClass=Auto  FilterContinuousStateAttributes=''  FilterStateMustResolveToSignalObject=off  FilterRTWStateStorageClass=Auto  DifferentiatorICPrevScaledInput=0  DifferentiatorOutMin=[]  DifferentiatorOutMax=[]
  PID Controller6 : simulink/Continuous/PID Controller  Controller=P  TimeDomain=Discrete-time  SampleTime=Tc  IntegratorMethod=Forward Euler  FilterMethod=Forward Euler  Form=Parallel  UseFilter=off  ControllerParametersSource=internal  P=1  I=35.1207902652377  D=0.2  N=40.0107970227961  InitialConditionSource=internal  InitialConditionForIntegrator=0  InitialConditionForFilter=0  ExternalReset=none  LimitOutput=off  UpperSaturationLimit=inf  LowerSaturationLimit=-inf  LinearizeAsGain=on  AntiWindupMode=none  Kb=1  TrackingMode=off  Kt=1  PParamMin=[]  PParamMax=[]  IParamMin=[]  IParamMax=[]  DParamMin=[]  DParamMax=[]  NParamMin=[]  NParamMax=[]  KbParamMin=[]  KbParamMax=[]  KtParamMin=[]  KtParamMax=[]  POutMin=[]  POutMax=[]  IOutMin=[]  IOutMax=[]  DOutMin=[]  DOutMax=[]  NOutMin=[]  NOutMax=[]  KbOutMin=[]  KbOutMax=[]  KtOutMin=[]  KtOutMax=[]  IntegratorOutMin=[]  IntegratorOutMax=[]  FilterOutMin=[]  FilterOutMax=[]  SumOutMin=[]  SumOutMax=[]  SumI1OutMin=[]  SumI1OutMax=[]  SumI2OutMin=[]  SumI2OutMax=[]  SumI3OutMin=[]  SumI3OutMax=[]  SumDOutMin=[]  SumDOutMax=[]  SaturationOutMin=[]  SaturationOutMax=[]  IntegratorContinuousStateAttributes=''  IntegratorStateMustResolveToSignalObject=off  IntegratorRTWStateStorageClass=Auto  FilterContinuousStateAttributes=''  FilterStateMustResolveToSignalObject=off  FilterRTWStateStorageClass=Auto  DifferentiatorICPrevScaledInput=0  DifferentiatorOutMin=[]  DifferentiatorOutMax=[]
  PID Controller7 : simulink/Continuous/PID Controller  Controller=PD  TimeDomain=Discrete-time  SampleTime=Tc  IntegratorMethod=Forward Euler  FilterMethod=Forward Euler  Form=Parallel  UseFilter=on  ControllerParametersSource=internal  P=-0.00239291827793903  I=0.005  D=-0.101936697537801  N=33.9318377685715  InitialConditionSource=internal  InitialConditionForIntegrator=0  InitialConditionForFilter=0  ExternalReset=none  LimitOutput=off  UpperSaturationLimit=inf  LowerSaturationLimit=-inf  LinearizeAsGain=on  AntiWindupMode=none  Kb=1  TrackingMode=off  Kt=1  PParamMin=[]  PParamMax=[]  IParamMin=[]  IParamMax=[]  DParamMin=[]  DParamMax=[]  NParamMin=[]  NParamMax=[]  KbParamMin=[]  KbParamMax=[]  KtParamMin=[]  KtParamMax=[]  POutMin=[]  POutMax=[]  IOutMin=[]  IOutMax=[]  DOutMin=[]  DOutMax=[]  NOutMin=[]  NOutMax=[]  KbOutMin=[]  KbOutMax=[]  KtOutMin=[]  KtOutMax=[]  IntegratorOutMin=[]  IntegratorOutMax=[]  FilterOutMin=[]  FilterOutMax=[]  SumOutMin=[]  SumOutMax=[]  SumI1OutMin=[]  SumI1OutMax=[]  SumI2OutMin=[]  SumI2OutMax=[]  SumI3OutMin=[]  SumI3OutMax=[]  SumDOutMin=[]  SumDOutMax=[]  SaturationOutMin=[]  SaturationOutMax=[]  IntegratorContinuousStateAttributes=''  IntegratorStateMustResolveToSignalObject=off  IntegratorRTWStateStorageClass=Auto  FilterContinuousStateAttributes=''  FilterStateMustResolveToSignalObject=off  FilterRTWStateStorageClass=Auto  DifferentiatorICPrevScaledInput=0  DifferentiatorOutMin=[]  DifferentiatorOutMax=[]
  Saturation{,1..3} (4 alike) : Saturate  UpperLimit=30000  LowerLimit=-30000
  Scope{1..4,6,9,11..13} (9 alike) : Scope
  Sum{1..5,7,9..11} (9 alike) : Sum  Inputs=|+-
  Switch{,1..8} (9 alike) : Switch  Criteria=u2 > Threshold
  To Workspace : ToWorkspace  VariableName=pitch_setpoint_model  SaveFormat=Structure With Time  SampleTime=-1
  To Workspace1 : ToWorkspace  VariableName=pitchrate_setpoint_model  SaveFormat=Structure With Time  SampleTime=-1
  To Workspace10 : ToWorkspace  VariableName=yaw_value_model  SaveFormat=Structure With Time  SampleTime=Tc
  To Workspace11 : ToWorkspace  VariableName=y_position_model  SaveFormat=Structure With Time  SampleTime=Tc
  To Workspace12 : ToWorkspace  VariableName=z_position_model  SaveFormat=Structure With Time  SampleTime=Tc
  To Workspace2 : ToWorkspace  VariableName=x_command_model  SaveFormat=Structure With Time  SampleTime=-1
  To Workspace3 : ToWorkspace  VariableName=roll_setpoint_model  SaveFormat=Structure With Time  SampleTime=Tc
  To Workspace4 : ToWorkspace  VariableName=rollrate_setpoint_model  SaveFormat=Structure With Time  SampleTime=Tc
  To Workspace5 : ToWorkspace  VariableName=y_command_model  SaveFormat=Structure With Time  SampleTime=Tq
  To Workspace6 : ToWorkspace  VariableName=z_command_model  SaveFormat=Structure With Time  SampleTime=Tc
  To Workspace7 : ToWorkspace  VariableName=yawrate_setpoint_model  SaveFormat=Structure With Time  SampleTime=Tc
  To Workspace8 : ToWorkspace  VariableName=yaw_command_model  SaveFormat=Structure With Time  SampleTime=Tc
  To Workspace9 : ToWorkspace  VariableName=x_position_model  SaveFormat=Structure With Time  SampleTime=Tc
  height_controlled : Outport
  y_controlled : Outport  Port=2
  x_controlled : Outport  Port=3
  yaw_controlled : Outport  Port=4
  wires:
  pitch_rate/1 -> Scope6/1, Sum4/2
  z_setpoint/1 -> Sum7/1
  x_position/1 -> Scope4/1, To Workspace9/1, Sum5/2
  PID Controller3/1 -> Sum4/1, To Workspace1/1
  PID Controller4/1 -> Sum3/1, To Workspace/1
  pitch/1 -> Gain/1, Sum3/2
  Gain/1 -> Scope9/1
  PID Controller2/1 -> Saturation/1
  PID Controller5/1 -> Saturation1/1
  Switch/1 -> PID Controller4/1
  Sum5/1 -> Switch/3
  From Workspace/1 -> Switch/1
  x_setpoint/1 -> Sum5/1
  Constant/1 -> Switch/2
  Switch1/1 -> PID Controller3/1
  Sum3/1 -> Switch1/3
  Constant1/1 -> Switch1/2
  Switch2/1 -> PID Controller5/1
  Constant2/1 -> Switch2/2
  Sum4/1 -> Switch2/3
  From Workspace2/1 -> Switch2/1
  From Workspace1/1 -> Switch1/1
  roll_rate/1 -> Scope11/1, Sum10/2
  y_position/1 -> To Workspace11/1, Scope12/1, Sum11/2
  PID Controller6/1 -> Sum10/1, To Workspace4/1
  PID Controller7/1 -> Sum9/1, To Workspace3/1
  roll/1 -> Gain2/1, Sum9/2
  Gain2/1 -> Scope13/1
  PID Controller12/1 -> Saturation2/1
  Switch3/1 -> PID Controller7/1
  Sum11/1 -> Switch3/3
  From Workspace3/1 -> Switch3/1
  y_setpoint/1 -> Sum11/1
  Constant3/1 -> Switch3/2
  Switch4/1 -> PID Controller6/1
  Sum9/1 -> Switch4/3
  Constant4/1 -> Switch4/2
  Switch5/1 -> PID Controller12/1
  Constant5/1 -> Switch5/2
  Sum10/1 -> Switch5/3
  From Workspace5/1 -> Switch5/1
  From Workspace4/1 -> Switch4/1
  Constant6/1 -> Switch6/2
  Switch6/1 -> PID Controller11/1
  Sum7/1 -> Switch6/3
  From Workspace6/1 -> Switch6/1
  PID Controller11/1 -> Saturation3/1
  Saturation1/1 -> x_controlled/1, To Workspace2/1
  Saturation2/1 -> y_controlled/1, To Workspace5/1
  Saturation3/1 -> To Workspace6/1, height_controlled/1
  Saturation/1 -> To Workspace8/1, yaw_controlled/1
  yaw/1 -> To Workspace10/1, Scope3/1, Sum1/2
  Sum1/1 -> Switch7/3
  From Workspace7/1 -> Switch7/1
  yaw_setpoint/1 -> Sum1/1
  Constant7/1 -> Switch7/2
  Switch7/1 -> PID Controller10/1
  yaw_rate/1 -> Gain1/1, Sum2/2
  Gain1/1 -> Scope1/1
  Sum2/1 -> Switch8/3
  Constant8/1 -> Switch8/2
  From Workspace8/1 -> Switch8/1
  Switch8/1 -> PID Controller2/1
  PID Controller10/1 -> To Workspace7/1, Sum2/1
  z_position/1 -> To Workspace12/1, Scope2/1, Sum7/2

== matlab function test_model/Actuation/Gravity

 ==
function E_Fg = gravity(m, g)

E_Fg = [0; 0; m*g];

== matlab function test_model/Actuation/Lbe





 ==
function E_ro  = linear_body_earth_conversion(B_vo, euler_angles)

euler_rates = zeros(3,1);
E_ro = zeros(3,1);

phi = euler_angles(1);
theta = euler_angles(2);
psi = euler_angles(3);

Leb = [cos(theta)*cos(psi), sin(phi)*sin(theta)*cos(psi)-cos(phi)*sin(psi), cos(phi)*sin(theta)*cos(psi)+sin(phi)*sin(psi); ...
       cos(theta)*sin(psi), sin(phi)*sin(theta)*sin(psi)+cos(phi)*cos(psi), cos(phi)*sin(theta)*sin(psi)-sin(phi)*cos(psi); ...
           -sin(theta)    ,                sin(phi)*cos(theta)            ,                 cos(phi)*cos(theta)           ];

E_ro = Leb * B_vo;

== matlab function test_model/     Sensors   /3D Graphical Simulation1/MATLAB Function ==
function y = eigenaxis_ucart(u)


if abs(u(1))< 0.0001
    u(1) = 0.0001;
end

if abs(u(2))< 0.0001
    u(2) = 0.0001;
end

if abs(u(3))< 0.0001
    u(3) = 0.0001;
end

u = [ -u(1); -u(2); u(3) ];% [Pitch, Yaw, Roll] 

C11 = cos(u(2))*cos(u(3));
C12 = cos(u(2))*sin(u(3));
C13 = -sin(u(2));
C21 = sin(u(1))*sin(u(2))*cos(u(3))-cos(u(1))*sin(u(3));
C22 = sin(u(1))*sin(u(2))*sin(u(3))+cos(u(1))*cos(u(3));
C23 = sin(u(1))*cos(u(2));
C31 = cos(u(1))*sin(u(2))*cos(u(3))+sin(u(1))*sin(u(3));
C32 = cos(u(1))*sin(u(2))*sin(u(3))-sin(u(1))*cos(u(3));
C33 = cos(u(1))*cos(u(2));
    
theta = acos(0.5*(C11+C22+C33-1));

e = [C23-C32; C31-C13; C12-C21]/(2*sin(theta));
    
y = [e; theta];

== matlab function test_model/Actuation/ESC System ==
function Vb_eff   = ESC(P, Pmin, Pmax, Vb)

P1 = P(1);
P2 = P(2);
P3 = P(3);
P4 = P(4);

% Define u_Pi for each of the rotors, limiting it to be greater than 0
% u_P0 = (rotor_0_duty_cycle/100 - Pmin) / (Pmax - Pmin);
% u_P1 = (rotor_1_duty_cycle/100 - Pmin) / (Pmax - Pmin);
% u_P2 = (rotor_2_duty_cycle/100 - Pmin) / (Pmax - Pmin);
% u_P3 = (rotor_3_duty_cycle/100 - Pmin) / (Pmax - Pmin);
u_P0 = (P1 - Pmin) / (Pmax - Pmin);
u_P1 = (P2 - Pmin) / (Pmax - Pmin);
u_P2 = (P3 - Pmin) / (Pmax - Pmin);
u_P3 = (P4 - Pmin) / (Pmax - Pmin);


% Determine the effective battery voltage from each ESC
Vb_eff_0 = u_P0 * Vb;
Vb_eff_1 = u_P1 * Vb;
Vb_eff_2 = u_P2 * Vb;
Vb_eff_3 = u_P3 * Vb;
    
Vb_eff = [Vb_eff_0, Vb_eff_1, Vb_eff_2, Vb_eff_3];

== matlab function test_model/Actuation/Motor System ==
function w_dot = motor(Vb_eff, w, Rm, Kv, Kq, Kd, If, Jreq)

% Define each motors effective battery voltage
Vb_eff_0 = Vb_eff(1);
Vb_eff_1 = Vb_eff(2);
Vb_eff_2 = Vb_eff(3);
Vb_eff_3 = Vb_eff(4);

% Determine the angular velocity of each rotor from feedback
w_0 = w(1);
w_1 = w(2);
w_2 = w(3);
w_3 = w(4);

% Determine angular acceleration of each rotor
w_0_dot = 1/(Jreq*Rm*Kq) * Vb_eff_0 - 1/(Jreq*Rm*Kq*Kv) * w_0 - 1/(Jreq*Kq)*If - (Kd/Jreq) * w_0^2;
w_1_dot = 1/(Jreq*Rm*Kq) * Vb_eff_1 - 1/(Jreq*Rm*Kq*Kv) * w_1 - 1/(Jreq*Kq)*If - (Kd/Jreq) * w_1^2;
w_2_dot = 1/(Jreq*Rm*Kq) * Vb_eff_2 - 1/(Jreq*Rm*Kq*Kv) * w_2 - 1/(Jreq*Kq)*If - (Kd/Jreq) * w_2^2;
w_3_dot = 1/(Jreq*Rm*Kq) * Vb_eff_3 - 1/(Jreq*Rm*Kq*Kv) * w_3 - 1/(Jreq*Kq)*If - (Kd/Jreq) * w_3^2;

w_dot = [w_0_dot, w_1_dot, w_2_dot, w_3_dot];

== matlab function test_model/Actuation/Rotor System







 ==
function [B_omega_dot, B_vo_dot]= rotor(w_dot, w, B_Fg, B_omega, B_vo, m, Kt, Kd, rhx, rhy, rhz, Jreq, Jxx, Jyy, Jzz)

% Create J vector
J = [Jxx,  0 ,  0 ; ...
      0 , Jyy,  0 ; ...
      0 ,  0 , Jzz;];

% Create r_hi vector
rh_0 = [-rhx; rhy; -rhz];
rh_1 = [rhx; rhy; -rhz];
rh_2 = [-rhx; -rhy; -rhz];
rh_3 = [rhx; -rhy; -rhz];

% Define vector from body frame origin to center of mass
br_oc = [0; 0; 0];

% Define 3x3 Identity Matrix
I = eye(3);

% Create gamma vectors
gamma_Ti = [0; 0; -1];
gamma_omega_03 = [0; 0; 1];  %Rotors 0 and 3 use this gamma_omega vector
gamma_omega_12 = [0; 0; -1]; %Rotors 1 and 2 use this gamma_omega vector

% Define angular velocities for each rotor
w_0 = w(1);
w_1 = w(2);
w_2 = w(3);
w_3 = w(4);

% Define angular acceleration for each rotor
w_0_dot = w_dot(1);
w_1_dot = w_dot(2);
w_2_dot = w_dot(3);
w_3_dot = w_dot(4);

% Define the rotor force in the z-direction from each rotor
B_Fr_0 = Kt * w_0 * w_0 * gamma_Ti;
B_Fr_1 = Kt * w_1 * w_1 * gamma_Ti;
B_Fr_2 = Kt * w_2 * w_2 * gamma_Ti;
B_Fr_3 = Kt * w_3 * w_3 * gamma_Ti;

% Sum up the rotor forces in the z-direction from each vector to get the
% total body force in the z-direction
B_Fr = B_Fr_0 + B_Fr_1 + B_Fr_2 + B_Fr_3;

% Define the in-plane drag and induced torque produced by each rotor
 B_Q_d0 = -1 * Kd * w_0 * w_0 * gamma_omega_03;
 B_Q_d1 = -1 * Kd * w_1 * w_1 * gamma_omega_12;
 B_Q_d2 = -1 * Kd * w_2 * w_2 * gamma_omega_12;
 B_Q_d3 = -1 * Kd * w_3 * w_3 * gamma_omega_03;

% Sum up the total in-plane drag and induced torque to get the total
% in-plane drag and induced torque on the body
B_Q_d = B_Q_d0 + B_Q_d1 + B_Q_d2 + B_Q_d3;

% Define the force lever arm torque created from the force produced by each
% rotor in the z-direction
B_Q_F0 = cross( rh_0, B_Fr_0 );
B_Q_F1 = cross( rh_1, B_Fr_1 );
B_Q_F2 = cross( rh_2, B_Fr_2 );
B_Q_F3 = cross( rh_3, B_Fr_3 );

B_Q_F = B_Q_F0 + B_Q_F1 + B_Q_F2 + B_Q_F3;

%Define the change in angular momentum torque produced by each rotor 
B_Q_L0 = -1 * Jreq * ( cross(B_omega, w_0 * gamma_omega_03) + w_0_dot * gamma_omega_03 );
B_Q_L1 = -1 * Jreq * ( cross(B_omega, w_1 * gamma_omega_12) + w_1_dot * gamma_omega_12 ); 
B_Q_L2 = -1 * Jreq * ( cross(B_omega, w_2 * gamma_omega_12) + w_2_dot * gamma_omega_12 ); 
B_Q_L3 = -1 * Jreq * ( cross(B_omega, w_3 * gamma_omega_03) + w_3_dot * gamma_omega_03 );

% Sum up the total change in angular momentum torque produced by each rotor
B_Q_L = B_Q_L0 + B_Q_L1 + B_Q_L2 + B_Q_L3;

% Define the total rotor system torque as the sum of the in-plane drag and
% induced torque, force lever arm torque, and change in angular momentum
% torques
B_Q = B_Q_d + B_Q_F + B_Q_L;

% Define the body forces in the z-direction from each vector to get the
% total body force in the z-direction
B_F = B_Fr + B_Fg; 

% Define the body frame linear velocities
B_vo_dot = (m*I)^(-1) * ( B_F - cross( B_omega, m*(B_vo + cross(B_omega, br_oc)) ) );

% Define the body frame angular velocities
B_omega_dot = J ^(-1) * ( B_Q - cross(B_omega, J * B_omega) - cross(br_oc, B_F) );

== matlab function test_model/Actuation/Aeb














 ==
function euler_rates = angular_body_earth_conversion(B_omega, euler_angles)

phi = euler_angles(1);
theta = euler_angles(2);

Aeb = [1, sin(phi)*tan(theta), cos(phi)*tan(theta); ...
       0,     cos(phi)       ,        -sin(phi)   ; ...
       0,  sin(phi)/cos(theta), cos(phi)/cos(theta)];

   
euler_rates = Aeb * B_omega;

== matlab function test_model/Actuation/Lbe

















 ==
function [B_Fg, B_g]  = linear_earth_body_conversion(E_Fg, euler_angles, m)

phi = euler_angles(1);
theta = euler_angles(2);
psi = euler_angles(3);

Lbe = [             cos(theta)*cos(psi)              ,          cos(theta)*sin(psi)                  ,     -sin(theta)    ; ...
       sin(phi)*sin(theta)*cos(psi)-cos(phi)*sin(psi), sin(phi)*sin(theta)*sin(psi)+cos(phi)*cos(psi), sin(phi)*cos(theta); ...
       cos(phi)*sin(theta)*cos(psi)+sin(phi)*sin(psi), cos(phi)*sin(theta)*sin(psi)-sin(phi)*cos(psi), cos(phi)*cos(theta)];

B_Fg = Lbe * E_Fg;

B_g = B_Fg/m;

== matlab function test_model/     Sensors   /Complimentary Filter







 ==
%function euler_angles_IMU  = complimentaryFilter(accel_pitch, accel_roll, euler_angles_gyro, prev_euler_angles_IMU)
function euler_angles_IMU  = complimentaryFilter(accel_pitch, accel_roll, euler_angles_gyro)

% LOOP_TIME = 5*10^-3;
% 
% prev_phi = prev_euler_angles_IMU(1);
% prev_theta = prev_euler_angles_IMU(2);
% 
% phi_dot_gyro = euler_angles_gyro(1);
% theta_dot_gyro = euler_angles_gyro(2);

% phi = 0.98 * ( prev_phi + phi_dot_gyro * LOOP_TIME ) + 0.02 * accel_roll;
% theta = 0.98 * ( prev_theta + theta_dot_gyro * LOOP_TIME) + 0.02 * accel_pitch;
k_gyro = 1; 
k_accel = 1-k_gyro; 

phi = k_gyro * ( euler_angles_gyro(1) ) + k_accel * accel_roll;
theta = k_gyro * ( euler_angles_gyro(2) ) + k_accel * accel_pitch;

euler_angles_IMU = [phi; theta];

== matlab function test_model/     Sensors   /IMU





/






 ==
function [accelReading,gyroReading] = idealIMU(B_vo_dot, B_vo, B_Omega, B_g, r_oc, g)
%#codegen

a = B_vo_dot + cross(B_Omega,B_vo) ; % body frame acceleration 

accelReading = (a - B_g)/g ; % accelerometer reading (ideal)

gyroReading = B_Omega ; % gyroscope reading (ideal) 

end

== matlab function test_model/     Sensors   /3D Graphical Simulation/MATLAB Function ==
function y = eigenaxis_ucart(u)


if abs(u(1))< 0.0001
    u(1) = 0.0001;
end

if abs(u(2))< 0.0001
    u(2) = 0.0001;
end

if abs(u(3))< 0.0001
    u(3) = 0.0001;
end

u = [ -u(1); -u(2); u(3) ];% [Pitch, Yaw, Roll] 

C11 = cos(u(2))*cos(u(3));
C12 = cos(u(2))*sin(u(3));
C13 = -sin(u(2));
C21 = sin(u(1))*sin(u(2))*cos(u(3))-cos(u(1))*sin(u(3));
C22 = sin(u(1))*sin(u(2))*sin(u(3))+cos(u(1))*cos(u(3));
C23 = sin(u(1))*cos(u(2));
C31 = cos(u(1))*sin(u(2))*cos(u(3))+sin(u(1))*sin(u(3));
C32 = cos(u(1))*sin(u(2))*sin(u(3))-sin(u(1))*cos(u(3));
C33 = cos(u(1))*cos(u(2));
    
theta = acos(0.5*(C11+C22+C33-1));

e = [C23-C32; C31-C13; C12-C21]/(2*sin(theta));
    
y = [e; theta];

== matlab function test_model/     Sensors   /Aeb









 ==
function euler_rates_IMU = angular_body_earth_conversion(gyro_reading, euler_angles_IMU)

phi = euler_angles_IMU(1);
theta = euler_angles_IMU(2);

Aeb = [1, sin(phi)*tan(theta), cos(phi)*tan(theta); ...
       0,     cos(phi)       ,        -sin(phi)   ; ...
       0,  sin(phi)/cos(theta), cos(phi)/cos(theta)];

   
euler_rates_IMU = Aeb * gyro_reading;

== matlab function test_model/     Sensors   /Calculate Pitch and Roll











1 ==
function [accel_pitch, accel_roll] = getPitchAndRoll(accel_reading, accel_roll_prev)

mag = norm(accel_reading);

x_accel = accel_reading(1)/mag;
y_accel = accel_reading(2)/mag;
z_accel = accel_reading(3)/mag;

accel_pitch = atan(x_accel/sqrt(y_accel^2 + z_accel^2));
%unwrapped_pitch = unwrap([accel_pitch_prev accel_pitch]);
%accel_pitch = unwrapped_pitch(2);

accel_roll = atan2( -y_accel,(sign(-z_accel)*sqrt(z_accel^2 + (1/100)*x_accel^2)) );
unwrapped_roll = unwrap([accel_roll_prev accel_roll]);
accel_roll = unwrapped_roll(2);

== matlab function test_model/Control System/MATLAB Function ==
function P  = signal_mixer(height_controlled, y_controlled, x_controlled, yaw_controlled)

controller_outputs = [ height_controlled; x_controlled; y_controlled; yaw_controlled ];
signal_mixer = [ 1, -1, -1, -1; ... 
                 1,  1, -1,  1; ...
                 1, -1,  1,  1; ...
                 1,  1,  1, -1 ];

% signal_mixer = [ 1,  1, -1, -1; ... 
%                  1, -1, -1,  1; ...
%                  1,  1,  1,  1; ...
%                  1, -1,  1, -1 ];

P = signal_mixer * controller_outputs;

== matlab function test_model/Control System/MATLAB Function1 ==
function [z_corr, y_cor, x_corr, yaw_corr, pid_y_out, pid_roll_out] = c_controller(set_x, set_y, set_z, set_yaw, ...
    cur_x, cur_y, cur_z, ...
    cur_phi, cur_theta, cur_psi, ...
    cur_phi_d, cur_theta_d, cur_psi_d, vrpn_id, Tc)

out_z = -1;
out_y = -1;
out_x = -1;
out_yaw = -1;
c_pid_y = -1;
c_pid_roll = -1;

coder.ceval('c_controller', vrpn_id, Tc, set_x, set_y, set_z, set_yaw, ...
                    cur_x, cur_y, cur_z, ...
                    cur_phi, cur_theta, cur_psi, ...
                    cur_phi_d, cur_theta_d, cur_psi_d, ...
                    coder.wref(out_z), coder.wref(out_y), coder.wref(out_x), coder.wref(out_yaw), ...
                    coder.wref(c_pid_y), coder.wref(c_pid_roll));

z_corr = out_z;
y_cor = out_y;
x_corr = out_x;
pid_y_out = c_pid_y;
pid_roll_out = c_pid_roll;
yaw_corr = out_yaw;
